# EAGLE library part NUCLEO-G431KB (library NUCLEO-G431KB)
Check availability
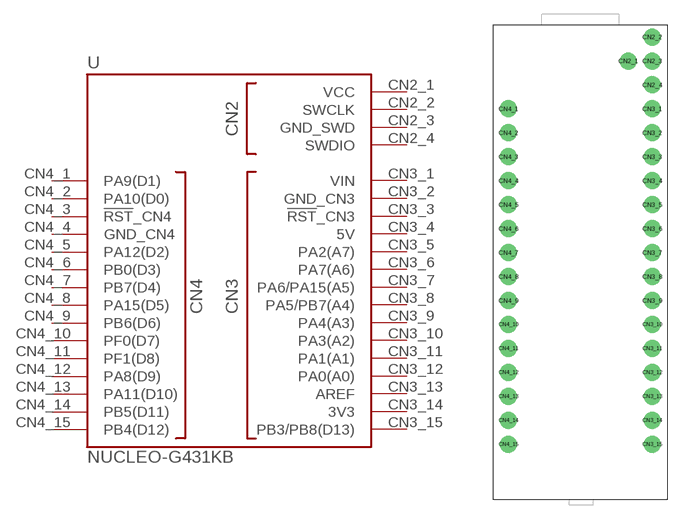
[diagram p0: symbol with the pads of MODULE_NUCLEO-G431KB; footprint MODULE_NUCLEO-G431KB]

Designator prefix U

## NUCLEO-G431KB (Availability: In Stock; Check_prices: https://www.snapeda.com/parts/NUCLEO-G431KB/STMicroelectronics/view-part/?ref=eda; Description: STM32G431 Nucleo-32 STM32G4 ARM® Cortex®-M4 MCU 32-Bit Embedded Evaluation Board; MF: STMicroelectronics; MP: NUCLEO-G431KB; Package: None; Price: None; SnapEDA_Link: https://www.snapeda.com/parts/NUCLEO-G431KB/STMicroelectronics/view-part/?ref=snap)  [MODULE_NUCLEO-G431KB]
CN2_1  VCC  pwr
CN2_2  SWCLK
CN2_3  GND_SWD  pwr
CN2_4  SWDIO
CN3_1  VIN  pwr
CN3_2  GND_CN3  pwr
CN3_3  !RST!_CN3  in
CN3_4  5V  pwr
CN3_5  PA2(A7)
CN3_6  PA7(A6)
CN3_7  PA6/PA15(A5)
CN3_8  PA5/PB7(A4)
CN3_9  PA4(A3)
CN3_10  PA3(A2)
CN3_11  PA1(A1)
CN3_12  PA0(A0)
CN3_13  AREF  pwr
CN3_14  3V3  pwr
CN3_15  PB3/PB8(D13)
CN4_1  PA9(D1)
CN4_2  PA10(D0)
CN4_3  !RST!_CN4  in
CN4_4  GND_CN4  pwr
CN4_5  PA12(D2)
CN4_6  PB0(D3)
CN4_7  PB7(D4)
CN4_8  PA15(D5)
CN4_9  PB6(D6)
CN4_10  PF0(D7)
CN4_11  PF1(D8)
CN4_12  PA8(D9)
CN4_13  PA11(D10)
CN4_14  PB5(D11)
CN4_15  PB4(D12)

## Footprint MODULE_NUCLEO-G431KB (pad centres in mm)
drill 1.2: CN2_1 5.08,21.336; CN2_2 7.62,23.876; CN2_3 7.62,21.336; CN2_4 7.62,18.796; CN3_1 7.62,16.256; CN3_2 7.62,13.716; CN3_3 7.62,11.176; CN3_4 7.62,8.636; CN3_5 7.62,6.096; CN3_6 7.62,3.556; CN3_7 7.62,1.016; CN3_8 7.62,-1.524; CN3_9 7.62,-4.064; CN3_10 7.62,-6.604; CN3_11 7.62,-9.144; CN3_12 7.62,-11.684; CN3_13 7.62,-14.224; CN3_14 7.62,-16.764; CN3_15 7.62,-19.304; CN4_1 -7.62,16.256; CN4_2 -7.62,13.716; CN4_3 -7.62,11.176; CN4_4 -7.62,8.636; CN4_5 -7.62,6.096; CN4_6 -7.62,3.556; CN4_7 -7.62,1.016; CN4_8 -7.62,-1.524; CN4_9 -7.62,-4.064; CN4_10 -7.62,-6.604; CN4_11 -7.62,-9.144; CN4_12 -7.62,-11.684; CN4_13 -7.62,-14.224; CN4_14 -7.62,-16.764; CN4_15 -7.62,-19.304

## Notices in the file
This work is licensed under a Creative Commons Attribution-ShareAlike 4.0 International License (CC BY-SA) with Design Exception 1.0
